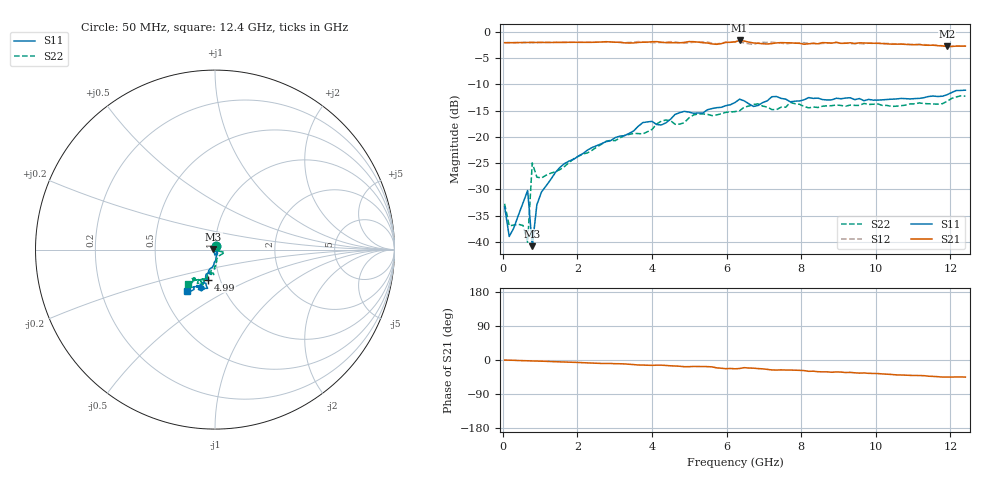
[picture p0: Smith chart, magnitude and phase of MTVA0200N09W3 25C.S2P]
! Network Analyzer HP8720D.06.14 Serial No. US36140669
! 24 Jul 2008  10:42:56
! Frequency  S11  S21  S12  S22
# HZ  S  DB R 50
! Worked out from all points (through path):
!   101 points, 50 MHz to 12.4 GHz, reference 50 ohm
!   highest |S21| = -1.66 dB at 6.348 GHz (marker M1); lowest = -2.8 dB at 11.91 GHz (marker M2)
!   group delay of S21, straight-line fit = 10.4 ps
!   lowest |S11| = -40.8 dB at 791 MHz (marker M3), VSWR 1.02, Z = 49.1 + j0.229 ohm
!   |S11| at or under -10 dB: start of sweep to end of sweep
!   |S22| runs from -40.1 to -12.2 dB; largest |S21 - S12| = 0.04
!   S11 on the Smith chart (normalised r, x): 50 MHz: 1.01, +0.04; 4.99 GHz: 0.88, -0.30; 12.4 GHz: 0.66, -0.33
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5e7  -33.31 74.2  -2.08 -0.3  -2.08 0.0  -32.74 70.1
1.735e8  -38.98 2.9  -2.07 -0.5  -2.08 -0.5  -36.96 13.8
5.44e8  -32.58 -71.0  -2.05 -1.7  -2.06 -1.6  -36.89 -37.2
6.675e8  -30.21 -90.9  -2.04 -2.0  -2.05 -2.0  -40.06 -31.4
7.91e8  -40.83 165.2  -2.03 -2.5  -2.06 -2.4  -24.97 -16.4
9.145e8  -32.92 -50.8  -2.04 -2.8  -2.06 -2.8  -27.68 -59.6
1.038e9  -30.52 -65.1  -2.02 -3.1  -2.04 -3.2  -27.84 -65.7
1.532e9  -25.83 -84.0  -2.03 -4.9  -2.02 -4.8  -26.25 -74.2
2.1495e9  -23.19 -92.1  -2.02 -7.1  -2.00 -7.0  -23.29 -82.3
3.755e9  -17.30 -103.8  -1.99 -13.3  -1.95 -12.0  -19.45 -94.3
4.249e9  -17.75 -104.2  -2.01 -13.6  -2.04 -14.8  -17.03 -97.2
4.743e9  -15.40 -106.3  -2.10 -16.5  -2.08 -15.6  -17.59 -99.2
4.99e9  -15.30 -102.6  -1.87 -17.6  -2.10 -17.9  -16.42 -106.8
6.225e9  -13.48 -110.4  -1.91 -23.2  -1.96 -21.3  -15.20 -110.1
6.3485e9  -12.84 -108.1  -1.66 -22.5  -1.87 -21.0  -15.04 -113.0
6.719e9  -14.22 -105.2  -2.14 -21.5  -2.44 -23.5  -13.84 -112.4
7.213e9  -12.37 -112.5  -2.26 -26.2  -1.99 -24.8  -14.82 -109.8
7.707e9  -13.34 -107.4  -2.11 -26.6  -2.19 -28.0  -13.44 -117.6
8.3245e9  -12.69 -110.8  -2.23 -29.5  -2.17 -29.0  -14.33 -117.0
1.0424e10  -12.84 -116.1  -2.36 -38.1  -2.27 -38.3  -14.23 -125.1
1.1906e10  -12.00 -117.8  -2.81 -45.0  -2.81 -44.8  -13.26 -124.7
1.24e10  -11.12 -124.6  -2.74 -45.2  -2.67 -44.9  -12.26 -128.8
